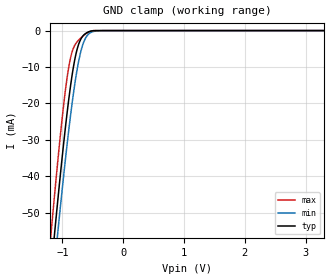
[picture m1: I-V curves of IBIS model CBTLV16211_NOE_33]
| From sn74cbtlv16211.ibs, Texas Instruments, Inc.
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[Model]   CBTLV16211_NOE_33
Model_type  Input
Vinl = 0.8
Vinh = 2.0
| variable   typ   min   max
C_comp   2.45pF   1.80pF   2.94pF
[Temperature Range]   40   100   -40
| Ambient temperature   25   85   -40
[Voltage range]   3.3   3   3.6
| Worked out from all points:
|   GND clamp passes 1 mA (typ) near -0.63 V on its own axis
[GND Clamp]
| CBTLV16211_NOE_33
|   Voltage   I(typ)   I(min)   I(max)
-3.3V     -497.5mA   -495.2mA   -503.4mA
-1.19V    -66.45mA   -74.91mA   -56.19mA
-1.135V   -56.72mA   -65.38mA   -46.15mA
-1.09V    -48.95mA   -57.75mA   -38.2mA
-1.065V   -44.73mA   -53.57mA   -33.92mA
-970mV    -29.48mA   -38.33mA   -19.01mA
-870mV    -15.62mA   -23.79mA   -7.765mA
-740mV    -4.1mA     -9.036mA   -2.718mA
-665mV    -1.521mA   -3.879mA   -1.552mA
-595mV    -554.8uA   -1.42mA    -660.7uA
-370mV    -2.165uA   -34.13uA   -40.97nA
3.3V      1.127nA    59.66nA    9.713pA
